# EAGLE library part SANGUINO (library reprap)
See http://www.sanguino.cc
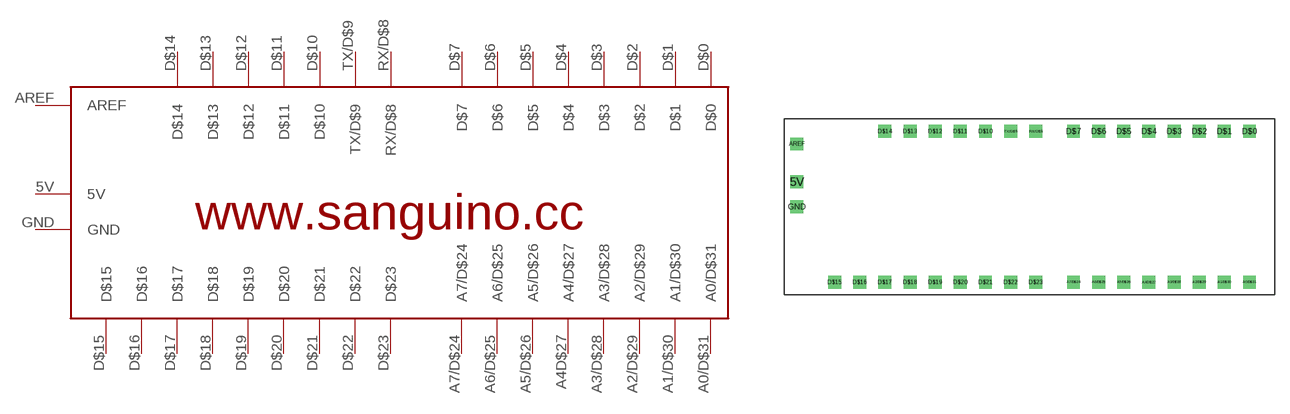
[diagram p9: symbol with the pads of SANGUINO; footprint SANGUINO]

Designator prefix -

## SANGUINO  [SANGUINO]
5V  5V  pwr
A0/D$31  A0/D$31
A1/D$30  A1/D$30
A2/D$29  A2/D$29
A3/D$28  A3/D$28
A4D$27  A4/D$27
A5/D$26  A5/D$26
A6/D$25  A6/D$25
A7/D$24  A7/D$24
AREF  AREF  out
D$0  D$0
D$1  D$1
D$2  D$2
D$3  D$3
D$4  D$4
D$5  D$5
D$6  D$6
D$7  D$7
D$10  D$10
D$11  D$11
D$12  D$12
D$13  D$13
D$14  D$14
D$15  D$15
D$16  D$16
D$17  D$17
D$18  D$18
D$19  D$19
D$20  D$20
D$21  D$21
D$22  D$22
D$23  D$23
GND  GND  pwr
RX/D$8  RX/D$8
TX/D$9  TX/D$9

## Footprint SANGUINO (pad centres in mm)
drill 0.8 square: 5V -22.86,3.81; A0/D$31 22.86,-6.35; A1/D$30 20.32,-6.35; A2/D$29 17.78,-6.35; A3/D$28 15.24,-6.35; A4D$27 12.7,-6.35; A5/D$26 10.16,-6.35; A6/D$25 7.62,-6.35; A7/D$24 5.08,-6.35; AREF -22.86,7.62; D$0 22.86,8.89; D$1 20.32,8.89; D$2 17.78,8.89; D$3 15.24,8.89; D$4 12.7,8.89; D$5 10.16,8.89; D$6 7.62,8.89; D$7 5.08,8.89; D$10 -3.81,8.89; D$11 -6.35,8.89; D$12 -8.89,8.89; D$13 -11.43,8.89; D$14 -13.97,8.89; D$15 -19.05,-6.35; D$16 -16.51,-6.35; D$17 -13.97,-6.35; D$18 -11.43,-6.35; D$19 -8.89,-6.35; D$20 -6.35,-6.35; D$21 -3.81,-6.35; D$22 -1.27,-6.35; D$23 1.27,-6.35; GND -22.86,1.27; RX/D$8 1.27,8.89; TX/D$9 -1.27,8.89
